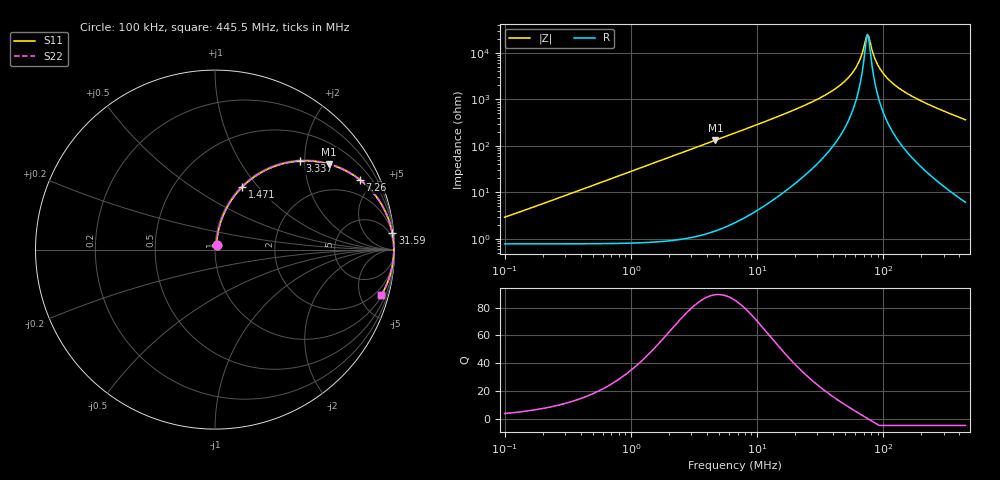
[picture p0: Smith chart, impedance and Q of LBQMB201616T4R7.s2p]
! LBQMB201616T4R7  S-PARAMETER MODEL  ( General Type )
! Model Generated by TAIYO YUDEN Corporation (http://www.ty-top.com)
! Version 1.0
! TAIYO YUDEN Control No. 191025NI43SB-FBB
! Copyright(c) 2019 TAIYO YUDEN CO.,LTD. All Rights Reserved.
! Product Description (link to TY-COMPAS)
! https://ds.yuden.co.jp/TYCOMPAS/or/detail?pn=LBQMB201616T4R7J&u=M
! Products Name : Inductors
! Characteristics :
!  Inductance : 4.7 uH , SRF(min) : 40 MHz , DC Resistance(max) : 1.014 Ohm , Rated Current : 270 mA
!  Case Size : 2.0 x 1.6 / 0.079 x 0.063 [mm/inch] , Thickness : 1.6 / 0.063 [mm/inch]
!  (Conditions: Temperature = 25 degC , DC Bias Current/Voltage = 0A / 0V)
! External Node Assignments :
!  1  o---GGG---o  2
! GND o---------o GND
! Frequency Range : 0.1MHz  -  445.549718MHz  [ 402 STEP ]
# MHz S RI R 50
! Freq[MHz].  S11 Real  S11 Imag  S21 Real  S21 Imag  S12 Real  S12 Imag  S22 Real  S22 Imag
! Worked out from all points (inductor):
!   401 points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, 100 kHz to 445.5 MHz, reference 50 ohm
!   read as one part in series: L = 4.5 uH near 104.3 kHz
!   highest Q = 89.4 at 4.671 MHz (marker M1), where L = 4.52 uH
!   self-resonance near 74.73 MHz
!   S11 on the Smith chart (normalised r, x): 100 kHz: 1.02, +0.06; 1.471 MHz: 1.02, +0.83; 3.337 MHz: 1.02, +1.89; 7.26 MHz: 1.05, +4.14; 31.59 MHz: 2, +22; 445.5 MHz: 1.12, -7.32
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0.1  0.00852 0.0278  0.9915 -0.0278  0.9915 -0.0278  0.00852 0.0278
0.408498  0.0207 0.1122  0.9793 -0.1122  0.9793 -0.1122  0.0207 0.1122
1.471116  0.1527 0.3496  0.8473 -0.3496  0.8473 -0.3496  0.1527 0.3496
1.668708  0.1867 0.3806  0.8133 -0.3806  0.8133 -0.3806  0.1867 0.3806
3.337445  0.4724 0.4933  0.5276 -0.4933  0.5276 -0.4933  0.4724 0.4933
4.670571  0.6359 0.4756  0.3641 -0.4756  0.3641 -0.4756  0.6359 0.4756
6.81664  0.7879 0.4029  0.2121 -0.4029  0.2121 -0.4029  0.7879 0.4029
7.260007  0.8082 0.3877  0.1918 -0.3877  0.1918 -0.3877  0.8082 0.3877
12.80081  0.9292 0.2481  0.0708 -0.2481  0.0708 -0.2481  0.9292 0.2481
27.26705  0.9836 0.1102  0.0164 -0.1102  0.0164 -0.1102  0.9836 0.1102
31.58594  0.9877 0.0905  0.0123 -0.0905  0.0123 -0.0905  0.9877 0.0905
44.20279  0.9933 0.0516  0.00668 -0.0516  0.00668 -0.0516  0.9933 0.0516
55.6922  0.9952 0.0281  0.00479 -0.0281  0.00479 -0.0281  0.9952 0.0281
64.51342  0.9958 0.014  0.00418 -0.014  0.00418 -0.014  0.9958 0.014
71.65744  0.996 0.00413  0.004 -0.00413  0.004 -0.00413  0.996 0.00413
74.73185  0.996 0.000191  0.00398 -0.000191  0.00398 -0.000191  0.996 0.000191
77.93817  0.996 -0.00375  0.004 0.00375  0.004 0.00375  0.996 -0.00375
84.76941  0.9959 -0.0116  0.00412 0.0116  0.00412 0.0116  0.9959 -0.0116
90.28298  0.9957 -0.0176  0.0043 0.0176  0.0043 0.0176  0.9957 -0.0176
111.3854  0.9945 -0.0381  0.00546 0.0381  0.00546 0.0381  0.9945 -0.0381
184.4005  0.9867 -0.0954  0.0133 0.0954  0.0133 0.0954  0.9867 -0.0954
445.5497  0.927 -0.252  0.073 0.252  0.073 0.252  0.927 -0.252
